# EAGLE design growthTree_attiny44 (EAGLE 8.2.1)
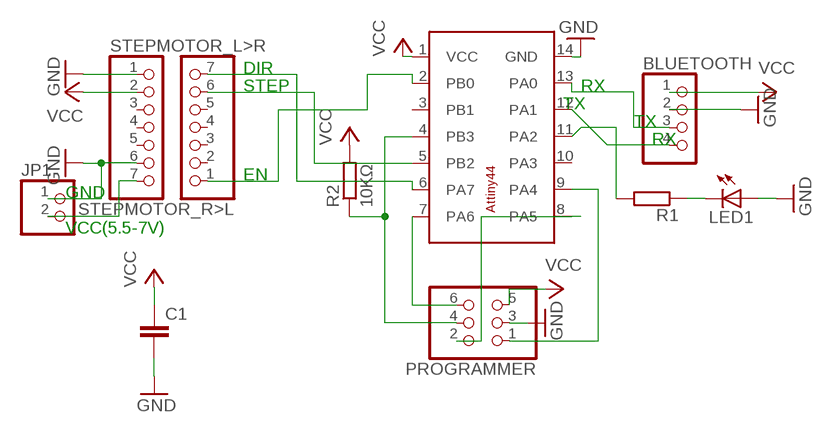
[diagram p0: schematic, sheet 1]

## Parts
BLUETOOTH  PINHD-1X4  [1X04]
C1  C-EUC1206  [C1206]
JP1  PINHD-1X2  [1X02]
LED1  LEDCHIPLED_1206  [CHIPLED_1206]
PROGRAMMER  PINHD-2X3  [2X03]
R1  R-EU_R1206  [R1206]
R2  10KΩ  R-EU_R1206  [R1206]
STEPMOTOR_L>R  PINHD-1X7  [1X07]
STEPMOTOR_R>L  PINHD-1X7  [1X07]
U$1  ATTINY44-SO14  [SO14]

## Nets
GND: BLUETOOTH.2 C1.2 JP1.1 LED1.A PROGRAMMER.3 STEPMOTOR_L>R.1 STEPMOTOR_L>R.6 U$1.14(GND)
MISO: PROGRAMMER.2 U$1.8(PA5)
MOSI: PROGRAMMER.6 U$1.7(PA6)
N$1: BLUETOOTH.3 U$1.13(PA0)
N$2: BLUETOOTH.4 U$1.12(PA1)
N$3: LED1.C R1.1
N$4: R1.2 U$1.11(PA2)
N$5: STEPMOTOR_R>L.7 U$1.6(PA7)
N$6: STEPMOTOR_R>L.6 U$1.5(PB2)
N$7: STEPMOTOR_R>L.1 U$1.2(PB0)
N$8: JP1.2 STEPMOTOR_L>R.7
RESET: PROGRAMMER.4 R2.1 U$1.4(PB3)
SCK: PROGRAMMER.1 U$1.9(PA4)
VCC: BLUETOOTH.1 C1.1 PROGRAMMER.5 R2.2 STEPMOTOR_L>R.2 U$1.1(VCC)
Unconnected: STEPMOTOR_L>R.3 STEPMOTOR_L>R.4 STEPMOTOR_L>R.5 STEPMOTOR_R>L.2 STEPMOTOR_R>L.3 STEPMOTOR_R>L.4 STEPMOTOR_R>L.5 U$1.3(PB1) U$1.10(PA3)

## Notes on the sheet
- DIR
- STEP | RX
- TX
- TX
- RX
- EN
- GND
- VCC(5.5-7V)

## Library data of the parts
BLUETOOTH = pinhead:PINHD-1X4: PIN HEADER
C1 = resistor:C-EU: CAPACITOR, European symbol
JP1 = pinhead:PINHD-1X2: PIN HEADER
LED1 = led:LED: LED
PROGRAMMER = pinhead:PINHD-2X3: PIN HEADER
R1 R2 = resistor:R-EU_: RESISTOR, European symbol
STEPMOTOR_L>R STEPMOTOR_R>L = pinhead:PINHD-1X7: PIN HEADER
U$1 = atmel-new:ATTINY44-SO14

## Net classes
0 default: width 0.61 mm

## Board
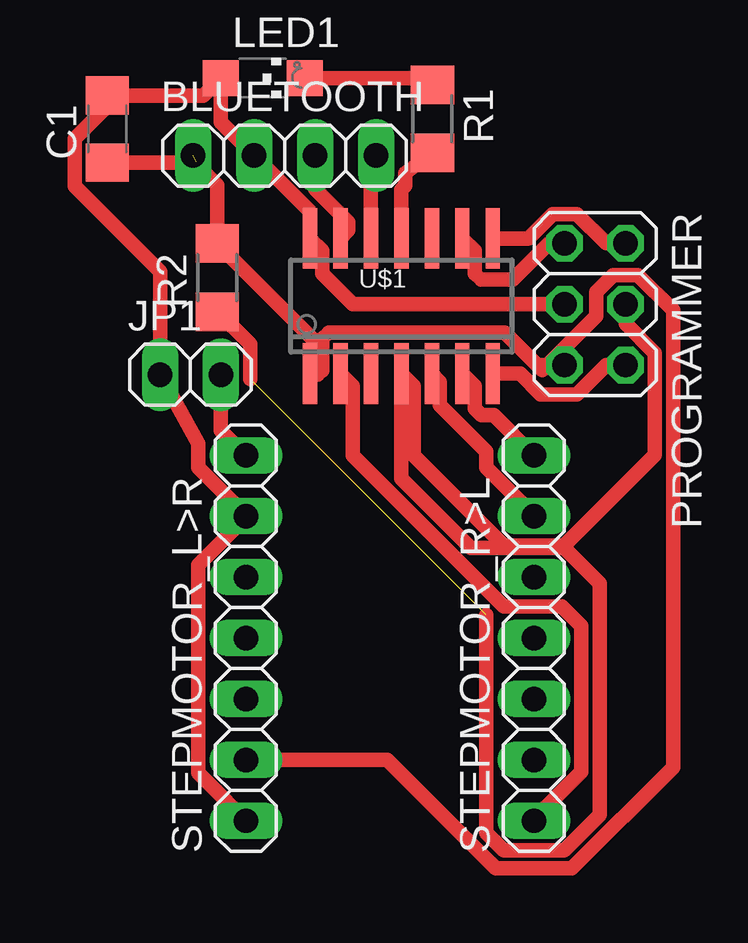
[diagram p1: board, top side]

No outline drawn. Coordinates in mm, seen from the top.
Copper layers (1*16): Top 0.035mm / dielectric 1.5mm / Bottom 0.035mm
Design rules "default": minimum track width 6mil, minimum drill 0.35mm, track to track 6mil, track to pad 6mil, pad to pad 6mil, via to via 6mil, smd to smd 6mil, copper to edge 40mil, drill to drill 6mil, minimum pad ring 10mil, minimum via ring 8mil, stop-mask expansion 4mil, vias tented up to drill 0mil, thermal gap 10mil

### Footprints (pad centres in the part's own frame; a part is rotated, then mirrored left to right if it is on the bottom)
1X04 = drill 1.016 long: 1 -3.81,0; 2 -1.27,0; 3 1.27,0; 4 3.81,0
C1206 = smd 1.6 x 1.8: 1 -1.4,0; 2 1.4,0
1X02 = drill 1.016 long: 1 -1.27,0; 2 1.27,0
CHIPLED_1206 = smd 1.5 x 1.5: A 0,-1.75; C 0,1.75
2X03 = drill 1.016 octagon: 1 -2.54,-1.27; 2 -2.54,1.27; 3 0,-1.27; 4 0,1.27; 5 2.54,-1.27; 6 2.54,1.27
R1206 = smd 1.6 x 1.803: 1 -1.422,0; 2 1.422,0
1X07 = drill 1.016 long: 1 -7.62,0; 2 -5.08,0; 3 -2.54,0; 4 0,0; 5 2.54,0; 6 5.08,0; 7 7.62,0
SO14 = smd 0.6 x 2.54: 1 -3.175,-2.822; 2 -1.905,-2.822; 3 -0.635,-2.822; 4 0.635,-2.822; 5 1.905,-2.822; 6 3.175,-2.822; 7 4.445,-2.822; 8 4.445,2.822; 9 3.175,2.822; 10 1.905,2.822; 11 0.635,2.822; 12 -0.635,2.822; 13 -1.905,2.822; 14 -3.175,2.822

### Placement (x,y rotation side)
BLUETOOTH  15.12,57.4 0 top
C1  7.73,58.5 90 top
JP1  11.2,48.26 0 top
LED1  14.21,60.63 270 top
PROGRAMMER  28.06,51.2 270 top
R1  21.28,58.92 270 top
R2  12.32,52.31 90 top
STEPMOTOR_L>R  13.51,37.28 90 top
STEPMOTOR_R>L  25.51,37.28 90 top
U$1  19.35,51.12 0 top

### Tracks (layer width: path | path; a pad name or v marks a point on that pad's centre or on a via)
GND
  Top 0.61: PROGRAMMER.3 17.97,51.2 16.69,52.48 16.69,53.43 U$1.14 16.18,55.08 BLUETOOTH.2 12.46,58.79 LED1.A 11.73,59.9 C1.2 7.73,59.45 6.37,58.09 6.37,56.11 9.93,52.55 JP1.1 11.53,45.39 11.53,44.4 13.51,42.41 STEPMOTOR_L>R.6 13.51,42.31 11.53,40.33 11.53,31.65 13.97,29.21 13.96,29.21 STEPMOTOR_L>R.1
MISO
  Top 0.61: PROGRAMMER.2 28.51,53.74 27.3,54.96 26.29,54.96 25.27,53.94 U$1.8
MOSI
  Top 0.61: PROGRAMMER.6 28.51,48.66 27.3,47.44 25.79,47.44 24.93,48.3 U$1.7
N$1
  Top 0.61: BLUETOOTH.3 16.39,56 17.78,54.61 17.78,54.28 U$1.13
N$2
  Top 0.61: U$1.12 18.71,57.19 BLUETOOTH.4
N$3
  Top 0.61: LED1.C 20.99,60.63 R1.1
N$4
  Top 0.61: U$1.11 19.98,55.97 20.15,56.13 20.15,56.67 R1.2
N$5
  Top 0.61: U$1.6 23.04,47.78 23.04,46.84 23.31,46.57 23.84,46.57 STEPMOTOR_R>L.7
N$6
  Top 0.61: STEPMOTOR_R>L.6 25.51,42.41 23.53,44.4 23.53,45.05 21.59,46.99 21.59,47.96 U$1.5
N$7
  Top 0.61: U$1.2 17.96,47.78 17.96,44.89 24.24,38.6 26.68,38.6 27.49,37.78 27.49,31.7 25.51,29.71 STEPMOTOR_R>L.1
N$8
  Top 0.61: JP1.2 12.47,45.94 STEPMOTOR_L>R.7
RESET  (1 unrouted)
  Top 0.61: PROGRAMMER.4 29.33,50.38 30.55,49.16 30.55,44.91 26.78,41.14 24.24,41.14 20.5,44.89 20.5,47.78 U$1.4 19.98,43.94 22.88,41.04 26.78,41.04 28.25,39.56 28.25,29.92 26.78,28.44 24.24,28.44 23.53,29.16 23.53,38.24 | R2.1 12.97,50.24 13.69,49.53 13.69,48.08
SCK
  Top 0.61: PROGRAMMER.1 26.14,53.74 24.62,52.22 23.31,52.22 23.04,52.48 23.04,53.43 U$1.9
VCC  (1 unrouted)
  Top 0.61: 16.69,49.76 16.96,50.02 | PROGRAMMER.5 25.65,48.66 24.28,50.02 | 16.69,49.76 16.69,48.81 U$1.1 | 24.28,50.02 16.96,50.02 | 11.38,57.1 C1.1 | 11.43,57.15 11.38,57.1 | 16.96,50.02 16.69,49.76 | 24.28,50.02 16.96,50.02 | 24.28,50.02 25.86,48.45 28.11,50.7 28.11,51.7 28.82,52.42 29.84,52.42 31.31,50.94 31.31,31.9 27.09,27.68 23.93,27.68 19.41,32.2 STEPMOTOR_L>R.2 | 16.69,49.76 16.68,49.75 16.68,48.43 16.51,48.26 16.51,49.54 R2.2 12.32,56.16 11.38,57.1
